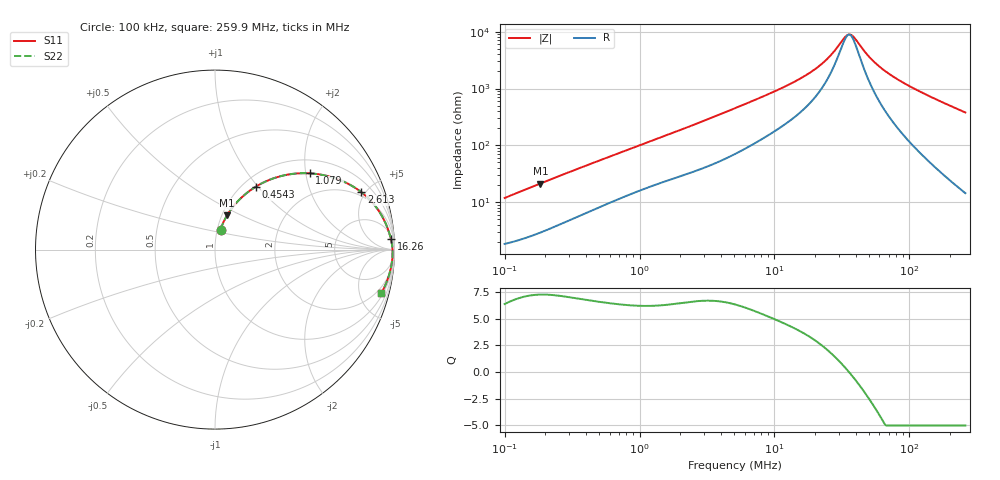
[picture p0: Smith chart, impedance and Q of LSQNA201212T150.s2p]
! LSQNA201212T150  S-PARAMETER MODEL  ( General Type )
! Model Generated by TAIYO YUDEN Corporation (http://www.ty-top.com)
! Version 2.0
! TAIYO YUDEN Control No. 100810NF25SB-FKC
! Copyright(c) 2007 TAIYO YUDEN CO.,LTD. All Rights Reserved.
! Product Description (link to TY-COMPAS)
! https://ds.yuden.co.jp/TYCOMPAS/or/detail?pn=LSQNA201212T150K&u=M
! Products Name : Inductors
! Characteristics :
!  Inductance : 15 uH , SRF(min) : 28 MHz , DC Resistance(max) : 1.69 Ohm
!  Rated Current : Saturation :170 mA , Temp Rise : 320 mA (40 degC)
!  Case Size : 2.0 x 1.25 / 0.079 x 0.049 [mm/inch] , Thickness : 1.25 / 0.049 [mm/inch]
!  (Conditions: Temperature = 25 degC , DC Bias Current/Voltage = 0A / 0V)
! External Node Assignments :
!  1  o---GGG---o  2
! GND o---------o GND
! Frequency Range : 0.1MHz  -  259.929867MHz  [ 402 STEP ]
# MHz S RI R 50
! Freq[MHz].  S11 Real  S11 Imag  S21 Real  S21 Imag  S12 Real  S12 Imag  S22 Real  S22 Imag
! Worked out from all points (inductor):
!   401 points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, 100 kHz to 259.9 MHz, reference 50 ohm
!   read as one part in series: L = 18.5 uH near 104 kHz
!   highest Q = 7.25 at 183.9 kHz (marker M1), where L = 18.2 uH
!   self-resonance near 35 MHz
!   S11 on the Smith chart (normalised r, x): 100 kHz: 1.04, +0.23; 454.3 kHz: 1.15, +0.97; 1.079 MHz: 1.34, +2.11; 2.613 MHz: 1.71, +4.70; 16.26 MHz: 9, +31; 259.9 MHz: 1.29, -7.56
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0.1  0.0308 0.1112  0.9692 -0.1112  0.9692 -0.1112  0.0308 0.1112
0.183929  0.0674 0.191  0.9326 -0.191  0.9326 -0.191  0.0674 0.191
0.37324  0.1776 0.3157  0.8224 -0.3157  0.8224 -0.3157  0.1776 0.3157
0.454318  0.2269 0.3503  0.7731 -0.3503  0.7731 -0.3503  0.2269 0.3503
0.714026  0.3724 0.4108  0.6276 -0.4108  0.6276 -0.4108  0.3724 0.4108
1.078932  0.5282 0.4248  0.4718 -0.4248  0.4718 -0.4248  0.5282 0.4248
1.393082  0.6235 0.4108  0.3765 -0.4108  0.3765 -0.4108  0.6235 0.4108
2.613156  0.8158 0.3194  0.1842 -0.3194  0.1842 -0.3194  0.8158 0.3194
5.098332  0.9248 0.1963  0.0752 -0.1963  0.0752 -0.1963  0.9248 0.1963
10.34583  0.9681 0.1007  0.0319 -0.1007  0.0319 -0.1007  0.9681 0.1007
16.25996  0.9803 0.0584  0.0197 -0.0584  0.0197 -0.0584  0.9803 0.0584
19.02902  0.9831 0.0458  0.0169 -0.0458  0.0169 -0.0458  0.9831 0.0458
24.56967  0.9864 0.0265  0.0136 -0.0265  0.0136 -0.0265  0.9864 0.0265
27.64535  0.9874 0.018  0.0126 -0.018  0.0126 -0.018  0.9874 0.018
32.99563  0.9886 0.00547  0.0114 -0.00547  0.0114 -0.00547  0.9886 0.00547
35.6948  0.9889 -0.000108  0.0111 0.000108  0.0111 0.000108  0.9889 -0.000108
38.61478  0.9892 -0.00572  0.0108 0.00572  0.0108 0.00572  0.9892 -0.00572
47.00293  0.9893 -0.0201  0.0107 0.0201  0.0107 0.0201  0.9893 -0.0201
53.93677  0.9891 -0.0306  0.0109 0.0306  0.0109 0.0306  0.9891 -0.0306
71.02397  0.9875 -0.0536  0.0125 0.0536  0.0125 0.0536  0.9875 -0.0536
120.7557  0.9781 -0.1105  0.0219 0.1105  0.0219 0.1105  0.9781 -0.1105
259.9299  0.9266 -0.2424  0.0734 0.2424  0.0734 0.2424  0.9266 -0.2424
